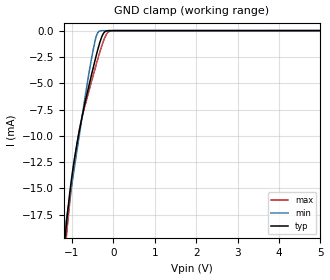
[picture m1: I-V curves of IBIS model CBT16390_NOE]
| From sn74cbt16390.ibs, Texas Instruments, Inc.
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[Model]   CBT16390_NOE
Model_type  Input
Vinl=0.8
Vinh=2.0
| variable   typ   min   max
C_comp   2.05pF   1.59pF   2.66pF
[Temperature Range]   40   100   -40
| Ambient temperature   25   85   -40
[Voltage range]   5   4.5   5.5
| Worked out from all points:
|   GND clamp passes 1 mA (typ) near -0.31 V on its own axis
[GND Clamp]
| CBT16390_NOE
|   Voltage   I(typ)   I(min)   I(max)
-5V       -229.8mA   -263mA     -210.9mA
-1.175V   -20.24mA   -19.19mA   -21.51mA
-1.15V    -19.18mA   -18.47mA   -20.41mA
-1.115V   -17.76mA   -17.55mA   -18.91mA
-950mV    -12.52mA   -13.34mA   -12.87mA
-800mV    -9.162mA   -9.452mA   -9.067mA
-485mV    -3.555mA   -1.836mA   -4.275mA
-405mV    -2.278mA   -482uA     -3.144mA
-335mV    -1.275mA   -40.43uA   -2.186mA
-165mV    -35.49uA   -9.428nA   -360.5uA
-20mV     -119nA     -10.11pA   -6.716uA
5V        333.5nA    125.5pA    4.468uA
